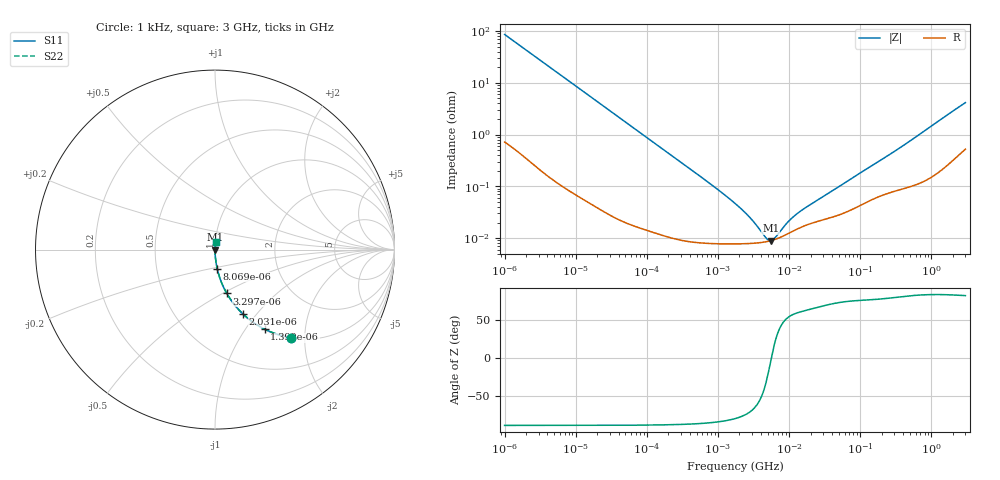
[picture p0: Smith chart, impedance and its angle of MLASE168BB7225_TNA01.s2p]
! MLASE168BB7225_TNA01  S-PARAMETER MODEL  ( Standard Model )
! Model Generated by TAIYO YUDEN Corporation (http://www.ty-top.com)
! Version 1.0
! TAIYO YUDEN Control No. 220601
! Copyright(c) 2012 TAIYO YUDEN CO.,LTD. All Rights Reserved.
! Product Description (link to TY-COMPAS)
! https://ds.yuden.co.jp/TYCOMPAS/or/detail?pn=MLASE168BB7225KTNA01&u=M
! Products Name : Multilayer Ceramic Capacitors
! Characteristics :
!  Capacitance : 2.2 [uF] , Rated Voltage : 16 [V] , TCC : X7R
!  Case Size : 1.6 x 0.8 / 0.063 x 0.031 [mm/inch] , Thickness : 0.8 / 0.031 [mm/inch]
!  (Conditions: Temperature = 25 [degC] , DC Bias Voltage = 0 [V])
! External Node Assignments :
!  1  o---| |---o  2
! GND o---------o GND
! Frequency Range : 1kHz  -  3GHz  [ 401 STEP ]
# MHZ S RI R 50
! Freq[MHz].  S11 Real  S11 Imag  S21 Real  S21 Imag  S12 Real  S12 Imag  S22 Real  S22 Imag
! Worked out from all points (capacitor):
!   401 points, 1 kHz to 3 GHz, reference 50 ohm
!   read as one part in series: C = 1.85 uF near 1.077 kHz
!   lowest |Z| = 8.93 mohm at 5.502 MHz (marker M1)
!   series resonance near 5.62 MHz, so ESL is about 430 pH
!   S11 on the Smith chart (normalised r, x): 1 kHz: 1.01, -1.72; 1.399 kHz: 1.01, -1.23; 2.031 kHz: 1.01, -0.85; 3.297 kHz: 1.00, -0.52; 8.069 kHz: 1.00, -0.22; 3 GHz: 1.01, +0.08
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0.001  0.4251 -0.4902  0.5749 0.4902  0.5749 0.4902  0.4251 -0.4902
0.001399  0.2763 -0.443  0.7237 0.443  0.7237 0.443  0.2763 -0.443
0.002031  0.1548 -0.3578  0.8452 0.3578  0.8452 0.3578  0.1548 -0.3578
0.003297  0.0659 -0.2444  0.9341 0.2444  0.9341 0.2444  0.0659 -0.2444
0.005158  0.0286 -0.1629  0.9714 0.1629  0.9714 0.1629  0.0286 -0.1629
0.008069  0.0122 -0.1061  0.9878 0.1061  0.9878 0.1061  0.0122 -0.1061
0.01216  0.00565 -0.071  0.9943 0.071  0.9943 0.071  0.00565 -0.071
0.033275  0.000946 -0.0262  0.9991 0.0262  0.9991 0.0262  0.000946 -0.0262
0.147855  0.000154 -0.00594  0.9998 0.00594  0.9998 0.00594  0.000154 -0.00594
0.762639  7.99e-05 -0.00114  0.9999 0.00114  0.9999 0.00114  7.99e-05 -0.00114
1.732051  7.74e-05 -0.000463  0.9999 0.000463  0.9999 0.000463  7.74e-05 -0.000463
2.812335  7.86e-05 -0.000236  0.9999 0.000236  0.9999 0.000236  7.86e-05 -0.000236
4.566395  8.42e-05 -6.56e-05  0.9999 6.56e-05  0.9999 6.56e-05  8.42e-05 -6.56e-05
4.919932  8.59e-05 -4.17e-05  0.9999 4.17e-05  0.9999 4.17e-05  8.59e-05 -4.17e-05
5.502215  8.91e-05 -6.54e-06  0.9999 6.54e-06  0.9999 6.54e-06  8.91e-05 -6.54e-06
6.387174  9.48e-05 3.98e-05  0.9999 -3.98e-05  0.9999 -3.98e-05  9.48e-05 3.98e-05
8.933959  0.000115 0.000143  0.9999 -0.000143  0.9999 -0.000143  0.000115 0.000143
11.1738  0.000135 0.000211  0.9999 -0.000211  0.9999 -0.000211  0.000135 0.000211
14.50609  0.00016 0.000293  0.9998 -0.000293  0.9998 -0.000293  0.00016 0.000293
21.06097  0.000195 0.000424  0.9998 -0.000424  0.9998 -0.000424  0.000195 0.000424
256.0921  0.000763 0.00401  0.9992 -0.00401  0.9992 -0.00401  0.000763 0.00401
3000  0.00685 0.0406  0.9932 -0.0406  0.9932 -0.0406  0.00685 0.0406
